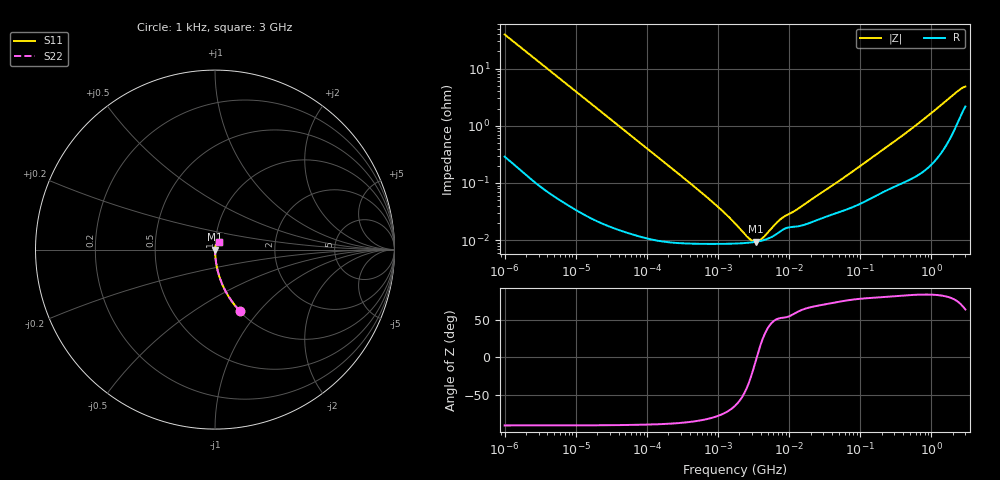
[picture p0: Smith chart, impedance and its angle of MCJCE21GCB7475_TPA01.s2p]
! MCJCE21GCB7475_TPA01  S-PARAMETER MODEL  ( Standard Model )
! Model Generated by TAIYO YUDEN Corporation (http://www.ty-top.com)
! Version 1.0
! TAIYO YUDEN Control No. 220601
! Copyright(c) 2015 TAIYO YUDEN CO.,LTD. All Rights Reserved.
! Product Description (link to TY-COMPAS)
! https://ds.yuden.co.jp/TYCOMPAS/or/detail?pn=MCJCE21GCB7475KTPA01&u=M
! Products Name : Multilayer Ceramic Capacitors
! Characteristics :
!  Capacitance : 4.7 [uF] , Rated Voltage : 16 [V] , TCC : X7R
!  Case Size : 2.0 x 1.25 / 0.079 x 0.049 [mm/inch] , Thickness : 1.25 / 0.049 [mm/inch]
!  (Conditions: Temperature = 25 [degC] , DC Bias Voltage = 0 [V])
! External Node Assignments :
!  1  o---| |---o  2
! GND o---------o GND
! Frequency Range : 1kHz  -  3GHz  [ 401 STEP ]
# MHZ S RI R 50
! Freq[MHz].  S11 Real  S11 Imag  S21 Real  S21 Imag  S12 Real  S12 Imag  S22 Real  S22 Imag
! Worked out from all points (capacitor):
!   401 points, 1 kHz to 3 GHz, reference 50 ohm
!   read as one part in series: C = 4.02 uF near 1.077 kHz
!   lowest |Z| = 9.35 mohm at 3.389 MHz (marker M1)
!   series resonance near 3.496 MHz, so ESL is about 520 pH
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0.001  0.1369 -0.3401  0.8631 0.3401  0.8631 0.3401  0.1369 -0.3401
0.001685  0.0538 -0.2221  0.9462 0.2221  0.9462 0.2221  0.0538 -0.2221
0.00306  0.0174 -0.1274  0.9826 0.1274  0.9826 0.1274  0.0174 -0.1274
0.005768  0.00524 -0.0686  0.9948 0.0686  0.9948 0.0686  0.00524 -0.0686
0.01216  0.00137 -0.0328  0.9986 0.0328  0.9986 0.0328  0.00137 -0.0328
0.147855  0.000104 -0.00272  0.9999 0.00272  0.9999 0.00272  0.000104 -0.00272
0.762639  8.6e-05 -0.000505  0.9999 0.000505  0.9999 0.000505  8.6e-05 -0.000505
1.192978  8.6e-05 -0.0003  0.9999 0.0003  0.9999 0.0003  8.6e-05 -0.0003
1.732051  8.69e-05 -0.000176  0.9999 0.000176  0.9999 0.000176  8.69e-05 -0.000176
2.709407  9e-05 -5.97e-05  0.9999 5.97e-05  0.9999 5.97e-05  9e-05 -5.97e-05
3.03007  9.14e-05 -3.32e-05  0.9999 3.32e-05  0.9999 3.32e-05  9.14e-05 -3.32e-05
3.388684  9.33e-05 -7.21e-06  0.9999 7.21e-06  0.9999 7.21e-06  9.33e-05 -7.21e-06
4.083148  9.77e-05 3.61e-05  0.9999 -3.61e-05  0.9999 -3.61e-05  9.77e-05 3.61e-05
7.696136  0.000145 0.000186  0.9999 -0.000186  0.9999 -0.000186  0.000145 0.000186
12.49624  0.000172 0.000288  0.9998 -0.000288  0.9998 -0.000288  0.000172 0.000288
21.06097  0.000207 0.000483  0.9998 -0.000483  0.9998 -0.000483  0.000207 0.000483
59.8242  0.000333 0.00121  0.9997 -0.00121  0.9997 -0.00121  0.000333 0.00121
256.0921  0.0008 0.00451  0.9992 -0.00451  0.9992 -0.00451  0.0008 0.00451
700.8126  0.00159 0.0116  0.9984 -0.0116  0.9984 -0.0116  0.00159 0.0116
2310.849  0.0122 0.0375  0.9878 -0.0375  0.9878 -0.0375  0.0122 0.0375
2682.519  0.018 0.041  0.982 -0.041  0.982 -0.041  0.018 0.041
3000  0.023 0.0413  0.977 -0.0413  0.977 -0.0413  0.023 0.0413
